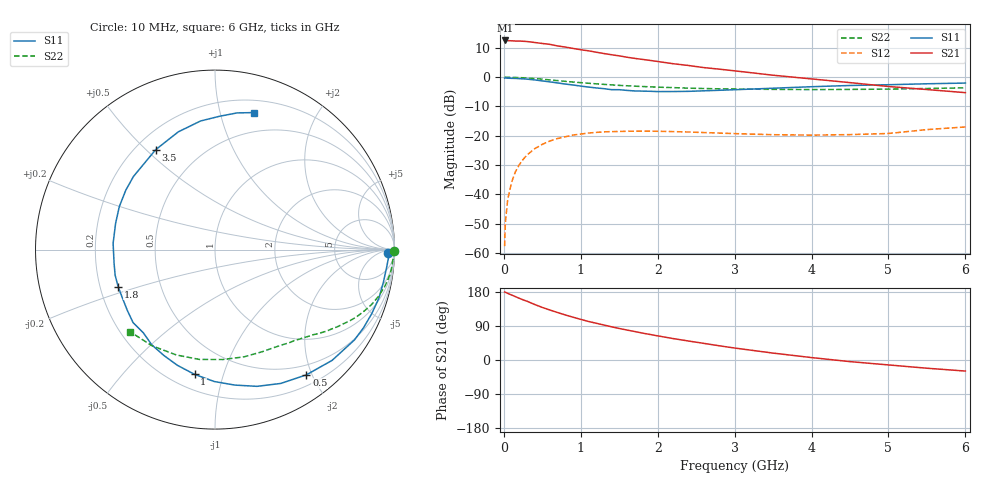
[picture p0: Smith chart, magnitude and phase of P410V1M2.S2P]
! SIEMENS Small Signal Semiconductors
! BFP182
! Si NPN RF Bipolar Junction Transistor in SOT143
! VCE = 10 V  IC = 1.2 mA
! Common Emitter S-Parameters:  March  1996
# GHz  S  MA  R  50
!  f  S11  S21  S12  S22
! GHz  MAG  ANG  MAG  ANG  MAG  ANG  MAG  ANG
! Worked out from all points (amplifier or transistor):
!   36 points, 10 MHz to 6 GHz, reference 50 ohm
!   highest |S21| = 12.5 dB at 20 MHz (marker M1)
!   |S21| within 3 dB of that: start of sweep to 961.5 MHz
!   unconditionally stable (mu >= 1): 2.561 GHz to end of sweep
!   at 250 MHz: K = 0.11, MSG = 20.2 dB, |S12| = -28.1 dB
!   at 1.4 GHz: K = 0.57, MSG = 13.1 dB, |S12| = -18.6 dB
!   at 6 GHz: K = 1.05, MAG = 4.5 dB, |S12| = -17.0 dB
!   S11 on the Smith chart (normalised r, x): 10 MHz: 44, -24; 500 MHz: 0.35, -1.92; 1 GHz: 0.29, -0.81; 1.8 GHz: 0.28, -0.17; 3.5 GHz: 0.28, +0.54; 6 GHz: 0.31, +1.28
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0.01  0.9651 -1.1  4.207 179.3  0.0013 81.3  0.9978 -0.4
0.02  0.9683 -2.3  4.237 178.8  0.0033 84.5  0.9983 -0.8
0.05  0.962 -5.6  4.205 175.8  0.0081 91.5  0.9955 -2.1
0.1  0.9555 -11.1  4.181 171.6  0.0159 82.6  0.9908 -4.2
0.15  0.9524 -16.6  4.142 167.3  0.0242 79.2  0.9888 -6.3
0.25  0.9353 -27.7  4.106 158.8  0.0394 72.6  0.9755 -10.4
0.3  0.9258 -32.9  4.064 155.2  0.0467 69.7  0.9674 -12.3
0.4  0.8981 -43.4  3.91 146.6  0.0599 63.3  0.9473 -16.0
0.5  0.8637 -53.9  3.762 138.7  0.0713 57.4  0.924 -19.4
0.6  0.831 -63.8  3.631 131.8  0.0814 51.8  0.898 -22.5
0.8  0.7628 -81.7  3.265 118.8  0.0961 42.2  0.8488 -27.9
1  0.7044 -99.3  2.939 107.2  0.1068 34.2  0.8064 -32.2
1.1  0.6779 -108.0  2.82 101.7  0.1112 30.8  0.7873 -34.1
1.4  0.6119 -130.7  2.417 87.6  0.1176 21.7  0.7391 -39.4
1.6  0.5946 -145.2  2.193 79.1  0.1192 17.3  0.7136 -42.4
1.8  0.5779 -159.1  2.014 71.1  0.12 13.8  0.693 -45.3
2.2  0.5687 176.5  1.698 56.6  0.1177 7.9  0.6634 -51.5
2.8  0.5972 146.3  1.371 37.5  0.111 3.3  0.6323 -61.3
3.5  0.6475 120.7  1.08 18.2  0.1041 2.7  0.6191 -74.8
4.5  0.7211 96.4  0.807 -4.3  0.1045 9.1  0.618 -98.0
5.5  0.7715 80.8  0.615 -21.7  0.1273 15.6  0.6406 -123.2
6  0.7933 74.2  0.544 -29.2  0.1413 14.5  0.6577 -135.8
